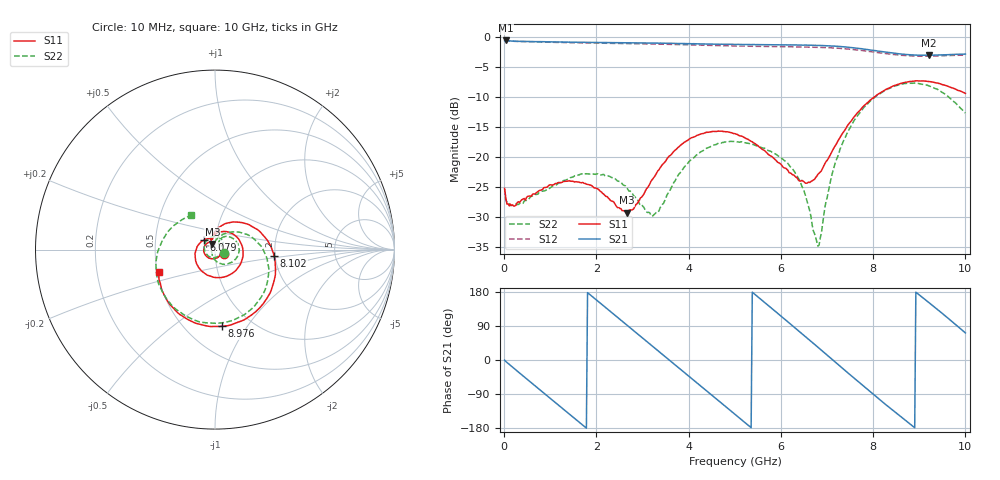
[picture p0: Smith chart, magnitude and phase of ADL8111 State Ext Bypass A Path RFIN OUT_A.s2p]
! Analog Devices Inc.
! Device:  ADL8111
! Description: Bypass Amplifier
! Frequency:  0.00 -  8.00 GHz
! Package:28-Lead Lead Frame Chip Scale Package[LFCSP] 6mm by 6mm
! Conditions:	Vdd = 5.0 V
!		State: External Bypass A
!		Path:  RFIN (Port1) to OUT_A (Port 2)
!		Idq = 70mA
!		Pin = -10 dBm
!		Temp = +25 C (baseplate temperature)
! Freq(Hz)	S11a(dB)	S11p(deg)	S21a(dB)	S21p(deg)	S12a(dB)	S12p(deg)	S22a(dB)	S22p(deg)
# Hz S  dB  R 50
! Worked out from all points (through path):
!   401 points, 10 MHz to 10 GHz, reference 50 ohm
!   highest |S21| = -0.63 dB at 34.98 MHz (marker M1); lowest = -3.1 dB at 9.201 GHz (marker M2)
!   group delay of S21, straight-line fit = 281 ps
!   lowest |S11| = -29.3 dB at 2.657 GHz (marker M3), VSWR 1.07, Z = 48.5 + j3.06 ohm
!   |S11| at or under -10 dB: start of sweep to 8.029 GHz
!   |S22| runs from -34.8 to -7.7 dB; largest |S21 - S12| = 0.033
!   S11 on the Smith chart (normalised r, x): 10 MHz: 1.10, -0.05; 6.079 GHz: 0.88, +0.10; 8.102 GHz: 1.97, -0.16; 8.976 GHz: 0.74, -0.78; 10 GHz: 0.51, -0.14
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1e7  -25.22 -24.2  -0.65 -0.4  -0.66 -0.1  -25.31 -18.6
3.4975e7  -26.73 -18.1  -0.63 -3.8  -0.66 -3.9  -27.19 -17.7
8.5915e8  -25.09 -113.3  -0.83 -87.2  -0.90 -87.2  -25.63 -143.2
1.233775e9  -24.25 -152.7  -0.88 -124.8  -0.96 -124.8  -24.18 165.1
1.683325e9  -24.26 162.8  -0.94 -169.8  -1.03 -169.8  -22.79 114.8
2.1079e9  -25.80 128.7  -0.99 147.7  -1.10 147.7  -22.96 73.8
2.65735e9  -29.25 114.1  -1.03 92.7  -1.16 92.6  -25.03 36.6
3.35665e9  -22.13 95.4  -1.09 22.4  -1.24 22.3  -28.95 54.5
3.781225e9  -18.35 55.0  -1.14 -20.4  -1.33 -20.5  -22.90 61.5
4.280725e9  -16.13 -1.6  -1.20 -70.7  -1.42 -70.7  -19.07 38.1
5.005e9  -16.12 -87.3  -1.30 -143.4  -1.55 -143.2  -17.43 -4.0
5.529475e9  -18.34 -153.4  -1.33 163.8  -1.61 164.0  -18.25 -30.7
6.078925e9  -21.82 137.9  -1.37 108.1  -1.68 108.4  -20.62 -60.4
6.678325e9  -23.95 103.0  -1.43 46.6  -1.75 47.1  -31.30 -128.2
6.828175e9  -22.70 99.6  -1.47 31.0  -1.78 31.6  -34.62 151.7
7.3027e9  -16.47 70.5  -1.65 -18.4  -1.96 -17.7  -18.28 51.5
7.727275e9  -12.13 30.1  -1.99 -62.5  -2.27 -61.6  -12.48 10.9
8.1019e9  -9.58 -6.4  -2.40 -100.5  -2.65 -99.6  -9.71 -23.9
8.35165e9  -8.51 -29.8  -2.64 -125.5  -2.89 -124.4  -8.60 -47.5
8.976025e9  -7.34 -84.6  -3.07 174.1  -3.24 175.0  -7.78 -106.4
9.2008e9  -7.44 -103.0  -3.10 152.2  -3.24 153.0  -8.16 -129.1
1e10  -9.42 -158.2  -2.90 71.4  -3.06 71.8  -12.68 124.9
